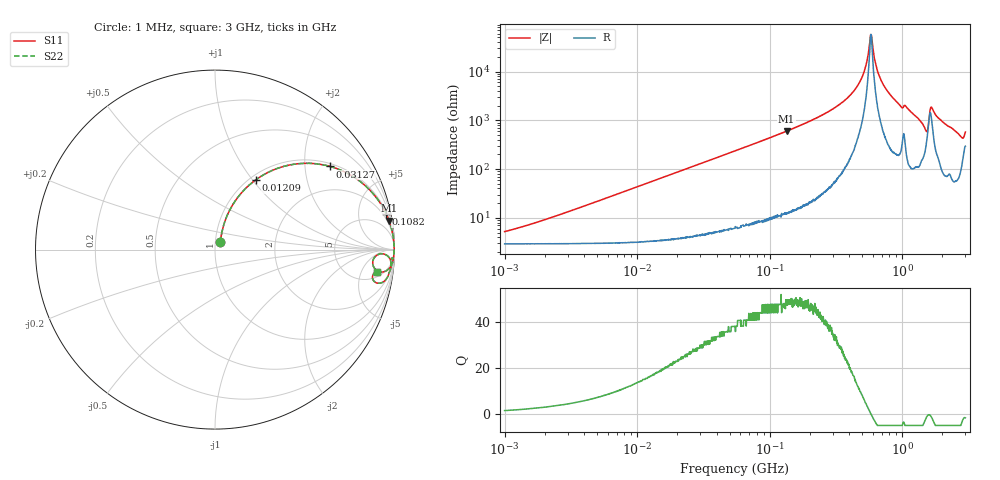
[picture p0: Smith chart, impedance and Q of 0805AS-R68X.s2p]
!s-Parameter Generated by FASTRON Sdn. Bhd.
!FASTRON P/N : 0805AS-R68X
!Keysight Technologies: E4991B_MY54100416_A.01.15
!Date: Mon Jun 15 12:55:48 2026
!Version  :Rev01  Mon Jun 15 12:55:48 2026
!Data & Calibration Information:
!Freq  S11  S21  S12  S22
!PortZ  Port1:50+j0  Port2:50+j0
!When reading reference impedance value at option line is always used.
! Remarks : This data is being provided solely for informational purposes.
# Hz S dB R 50
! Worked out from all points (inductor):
!   1601 points, 1 MHz to 3 GHz, reference 50 ohm
!   read as one part in series: L = 688 nH near 2.045 MHz
!   highest Q = 49.8 at 134.1 MHz (marker M1), where L = 711 nH
!   self-resonance near 581.2 MHz
!   S11 on the Smith chart (normalised r, x): 1 MHz: 1.06, +0.09; 12.09 MHz: 1.07, +1.04; 31.27 MHz: 1.09, +2.69; 108.2 MHz: 1.21, +9.52; 3 GHz: 7, -10
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1000000  -25.90 53.5  -0.26 -2.4  -0.26 -2.4  -25.90 53.5
3804036  -15.90 70.7  -0.36 -9.1  -0.36 -9.1  -15.90 70.7
1.20852e7  -6.91 59.6  -1.26 -26.8  -1.26 -26.8  -6.91 59.6
1.447069e7  -5.73 55.8  -1.64 -31.1  -1.64 -31.1  -5.73 55.8
3.127247e7  -2.05 35.9  -4.62 -52.1  -4.62 -52.1  -2.05 35.9
5.504702e7  -0.79 22.6  -8.29 -65.8  -8.29 -65.8  -0.79 22.6
1.081723e8  -0.23 11.8  -13.80 -76.9  -13.80 -76.9  -0.23 11.8
1.341416e8  -0.15 9.4  -15.70 -79.4  -15.70 -79.4  -0.15 9.4
2.083556e8  -0.06 5.7  -20.10 -83.1  -20.10 -83.1  -0.06 5.7
3.318279e8  -0.02 2.8  -26.30 -85.3  -26.30 -85.3  -0.02 2.8
4.391493e8  -0.02 1.4  -32.60 -84.9  -32.60 -84.9  -0.02 1.4
5.128394e8  -0.01 0.6  -39.50 -80.9  -39.50 -80.9  -0.01 0.6
5.81181e8  -0.01 0.0  -55.20 -2.8  -55.20 -2.8  -0.01 0.0
5.959055e8  -0.01 -0.1  -51.60 49.7  -51.60 49.7  -0.01 -0.1
6.296259e8  -0.02 -0.4  -43.30 74.8  -43.30 74.8  -0.02 -0.4
6.652545e8  -0.02 -0.7  -38.80 80.1  -38.80 80.1  -0.02 -0.7
7.925923e8  -0.02 -1.6  -31.30 83.8  -31.30 83.8  -0.02 -1.6
1.496395e9  -0.57 -7.7  -16.80 60.0  -16.80 60.0  -0.57 -7.7
1.67892e9  -0.24 -2.7  -25.30 58.2  -25.30 58.2  -0.24 -2.7
1.931433e9  -0.14 -5.4  -20.50 77.9  -20.50 77.9  -0.14 -5.4
2.75535e9  -0.50 -11.3  -14.00 68.2  -14.00 68.2  -0.50 -11.3
3e9  -0.82 -7.8  -16.00 51.3  -16.00 51.3  -0.82 -7.8
